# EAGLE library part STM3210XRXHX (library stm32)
ST STM32F 64 pin TFBGA
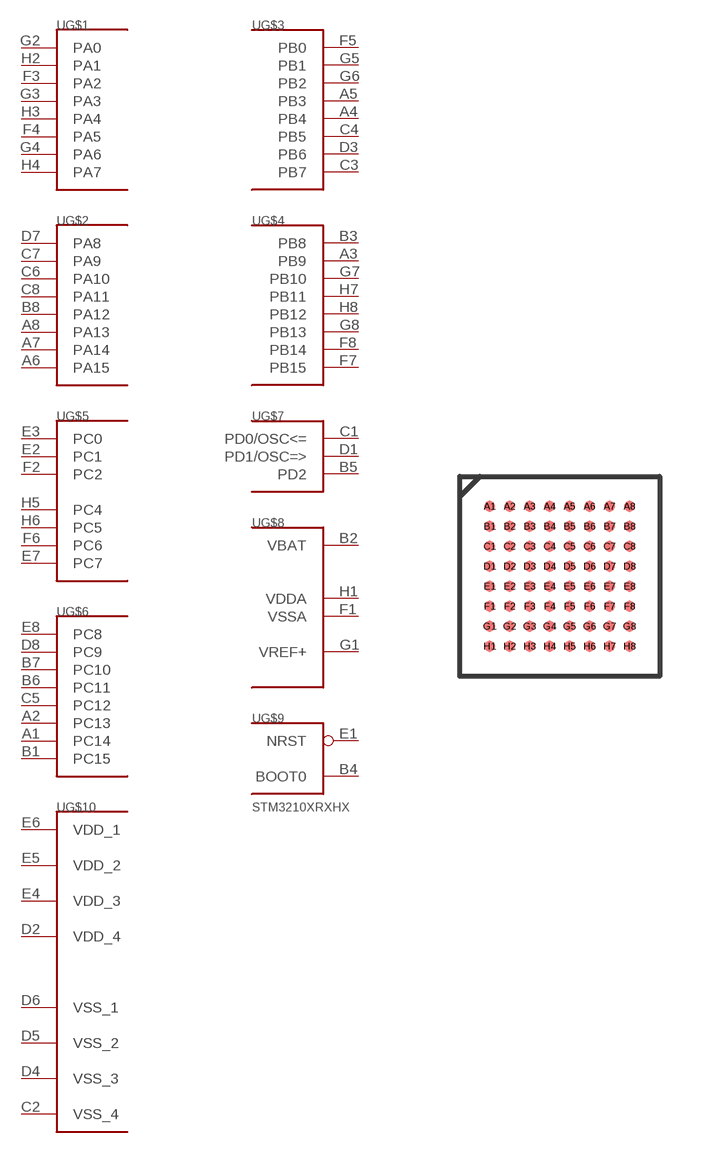
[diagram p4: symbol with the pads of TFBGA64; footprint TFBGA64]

Designator prefix U; gates G$1=PORT_A_L G$2=PORT_A_H G$3=PORT_B_L G$4=PORT_B_H G$5=PORT_C_NOPC3 G$6=PORT_C_H G$7=PORT_D_3 G$9=BOOT_RST G$10=VCC_VDD_M G$8=BAT_AN_NOVREF-

## STM3210XRXHX  [TFBGA64]
A1  G$6:PC14
A2  G$6:PC13
A3  G$4:PB9
A4  G$3:PB4
A5  G$3:PB3
A6  G$2:PA15
A7  G$2:PA14
A8  G$2:PA13
B1  G$6:PC15
B2  G$8:VBAT  pwr
B3  G$4:PB8
B4  G$9:BOOT0  in
B5  G$7:PD2
B6  G$6:PC11
B7  G$6:PC10
B8  G$2:PA12
C1  G$7:PD0/OSC<=
C2  G$10:VSS_4  pwr
C3  G$3:PB7
C4  G$3:PB5
C5  G$6:PC12
C6  G$2:PA10
C7  G$2:PA9
C8  G$2:PA11
D1  G$7:PD1/OSC=>
D2  G$10:VDD_4  pwr
D3  G$3:PB6
D4  G$10:VSS_3  pwr
D5  G$10:VSS_2  pwr
D6  G$10:VSS_1  pwr
D7  G$2:PA8
D8  G$6:PC9
E1  G$9:NRST  in
E2  G$5:PC1
E3  G$5:PC0
E4  G$10:VDD_3  pwr
E5  G$10:VDD_2  pwr
E6  G$10:VDD_1  pwr
E7  G$5:PC7
E8  G$6:PC8
F1  G$8:VSSA  pwr
F2  G$5:PC2
F3  G$1:PA2
F4  G$1:PA5
F5  G$3:PB0
F6  G$5:PC6
F7  G$4:PB15
F8  G$4:PB14
G1  G$8:VREF+  in
G2  G$1:PA0
G3  G$1:PA3
G4  G$1:PA6
G5  G$3:PB1
G6  G$3:PB2
G7  G$4:PB10
G8  G$4:PB13
H1  G$8:VDDA  pwr
H2  G$1:PA1
H3  G$1:PA4
H4  G$1:PA7
H5  G$5:PC4
H6  G$5:PC5
H7  G$4:PB11
H8  G$4:PB12

## Footprint TFBGA64 (pad centres in mm)
64 Ball TFBGA64 0.5mm pitch
smd 0.27 x 0.27: A1 -1.25,1.75; A2 -0.75,1.75; A3 -0.25,1.75; A4 0.25,1.75; A5 0.75,1.75; A6 1.25,1.75; A7 1.75,1.75; A8 2.25,1.75; B1 -1.25,1.25; B2 -0.75,1.25; B3 -0.25,1.25; B4 0.25,1.25; B5 0.75,1.25; B6 1.25,1.25; B7 1.75,1.25; B8 2.25,1.25; C1 -1.25,0.75; C2 -0.75,0.75; C3 -0.25,0.75; C4 0.25,0.75; C5 0.75,0.75; C6 1.25,0.75; C7 1.75,0.75; C8 2.25,0.75; D1 -1.25,0.25; D2 -0.75,0.25; D3 -0.25,0.25; D4 0.25,0.25; D5 0.75,0.25; D6 1.25,0.25; D7 1.75,0.25; D8 2.25,0.25; E1 -1.25,-0.25; E2 -0.75,-0.25; E3 -0.25,-0.25; E4 0.25,-0.25; E5 0.75,-0.25; E6 1.25,-0.25; E7 1.75,-0.25; E8 2.25,-0.25; F1 -1.25,-0.75; F2 -0.75,-0.75; F3 -0.25,-0.75; F4 0.25,-0.75; F5 0.75,-0.75; F6 1.25,-0.75; F7 1.75,-0.75; F8 2.25,-0.75; G1 -1.25,-1.25; G2 -0.75,-1.25; G3 -0.25,-1.25; G4 0.25,-1.25; G5 0.75,-1.25; G6 1.25,-1.25; G7 1.75,-1.25; G8 2.25,-1.25; H1 -1.25,-1.75; H2 -0.75,-1.75; H3 -0.25,-1.75; H4 0.25,-1.75; H5 0.75,-1.75; H6 1.25,-1.75; H7 1.75,-1.75; H8 2.25,-1.75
